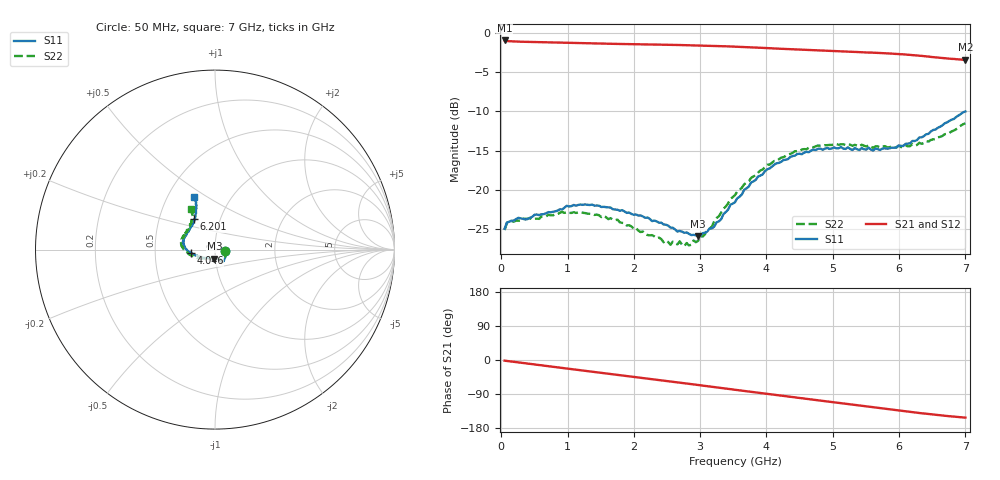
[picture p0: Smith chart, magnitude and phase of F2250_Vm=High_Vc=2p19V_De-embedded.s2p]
! Integrated Device Technology
! Corporate Headquarters
! 6024 Silver Creek Valley Road
! San Jose, CA 95138  USA
! Phone:  1-408-284-8200
! Toll Free:  1-800-223-1366
! Webpage:  http://www.idt.com/
! Timing and RF Division
! 515 Groton Road, Suite 102
! Westford, MA 01886-6024
! Device:  F2250
! Description: Voltage Variable RF Attenuator
! Frequency:  50.0 -  6000.00 MHz
! Package:  3x3 mm Thin QFN Plastic Package: 16 pin
! Ports:  2 RF, 3 DC
!  Pin  1  = GND
!  Pin  2  = NC
!  Pin  3  = RF1  = Port 1
!  Pin  4  = NC
!  Pin  5  = GND
!  Pin  6  = GND
!  Pin  7  = GND
!  Pin  8  = GND
!  Pin  9  = NC
!  Pin 10  = RF2  = Port 2
!  Pin 11  = NC
!  Pin 12  = GND
!  Pin 13  = GND
!  Pin 14  = VCNTRL
!  Pin 15  = VDD
!  Pin 16  = VMODE
! Vcntrl:  2.190 Volts
! Vmode:  +3.300 Volts
! Vdd:  +3.30  Volts
! Current:  1.317 mA
! Data:  The device was measured on a the F2250 evaluation board which has
!  individual transmission lines to the RF pins.  Data was collected
!  using a calibrated network analyzer.  The evaluation board was
!  de-embedded using a TRL calibration technique.
!  The reference plane is the edge of the package pin.
! Misc:  SN 10
!  Action Tracker AT0258
! Date Measured:  2014-11-26
! Date:  2015-10-15  MJV
! Note:
!  Integrated Device Technology supplies this data as a sample of measured
!  data at the package pin for this product.  Your particular data for this
!  product may vary.
!  Data was taken at 25 degrees C.
!  Integrated Device Technology reserves the right to change this data at anytime.
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# GHz S dB R 50
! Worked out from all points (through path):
!   201 points, 50 MHz to 7 GHz, reference 50 ohm
!   highest |S21| = -0.93 dB at 50 MHz (marker M1); lowest = -3.4 dB at 7 GHz (marker M2)
!   group delay of S21, straight-line fit = 61.1 ps
!   lowest |S11| = -25.9 dB at 2.969 GHz (marker M3), VSWR 1.11, Z = 49.4 - j4.99 ohm
!   |S11| at or under -10 dB: start of sweep to end of sweep
!   |S22| runs from -27.2 to -11.5 dB; largest |S21 - S12| = 0.0019
!   S11 on the Smith chart (normalised r, x): 50 MHz: 1.12, -0.02; 4.046 GHz: 0.76, -0.03; 6.201 GHz: 0.75, +0.27; 7 GHz: 0.68, +0.44
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0.05  -24.97 -9.9  -0.93 -1.8  -0.93 -1.8  -25.16 -10.3
0.1195  -24.08 -9.6  -1.03 -3.2  -1.03 -3.2  -24.06 -8.5
0.91875  -22.53 -48.0  -1.22 -21.0  -1.22 -21.1  -22.84 -49.7
1.2315  -21.93 -55.7  -1.28 -27.9  -1.28 -27.9  -22.95 -60.2
1.75275  -22.56 -62.6  -1.38 -39.1  -1.37 -39.1  -23.82 -67.1
2.37825  -24.22 -62.6  -1.47 -52.8  -1.47 -52.8  -26.11 -67.9
2.552  -24.84 -67.3  -1.49 -56.6  -1.49 -56.7  -27.03 -74.4
2.691  -25.27 -74.8  -1.52 -59.7  -1.52 -59.8  -26.60 -81.8
2.7605  -25.50 -76.9  -1.53 -61.3  -1.53 -61.3  -27.21 -86.2
2.969  -25.94 -93.8  -1.57 -66.0  -1.57 -66.0  -26.53 -104.7
3.21225  -24.71 -123.5  -1.63 -71.4  -1.62 -71.5  -24.00 -129.2
3.4555  -21.92 -145.2  -1.70 -76.9  -1.70 -77.0  -21.20 -144.5
3.525  -21.60 -149.6  -1.72 -78.5  -1.72 -78.5  -20.69 -147.8
3.76825  -19.07 -162.5  -1.81 -84.0  -1.81 -84.0  -18.49 -158.9
4.04625  -17.29 -172.3  -1.93 -90.2  -1.92 -90.2  -16.79 -169.4
4.4285  -15.65 177.4  -2.07 -98.6  -2.08 -98.6  -15.08 179.2
4.7065  -14.87 170.4  -2.17 -104.8  -2.17 -104.8  -14.58 173.4
5.054  -14.72 162.1  -2.30 -112.5  -2.30 -112.5  -14.18 166.3
5.85325  -14.72 136.1  -2.60 -130.0  -2.60 -130.1  -14.59 147.5
6.20075  -13.77 124.4  -2.81 -137.7  -2.81 -137.8  -14.18 138.4
6.54825  -12.32 116.3  -3.08 -144.7  -3.08 -144.8  -13.52 127.0
7  -10.01 111.3  -3.41 -152.1  -3.42 -152.2  -11.51 120.8
